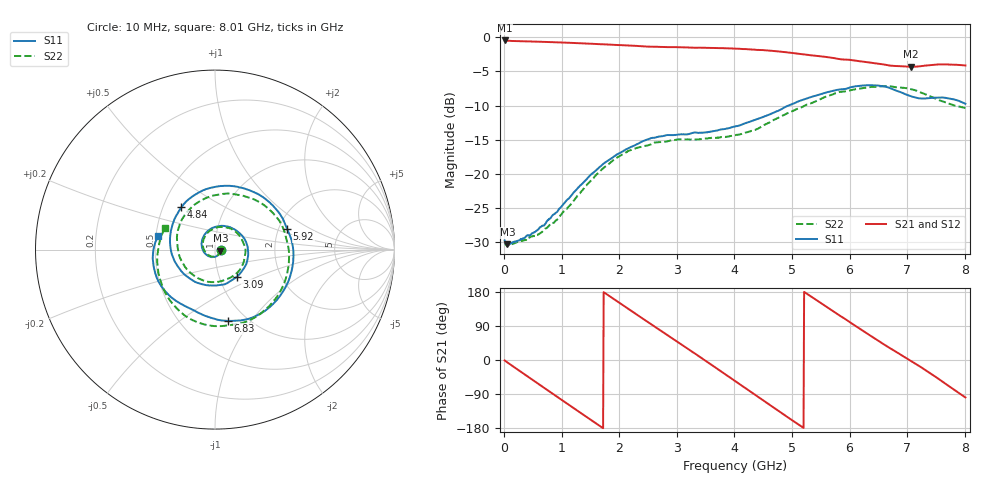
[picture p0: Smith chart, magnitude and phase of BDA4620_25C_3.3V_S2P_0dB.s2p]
!Agilent Technologies,E5071B,MY42404982,A.09.10
!Date: Wed May 06 08:55:57 2026
!Data & Calibration Information:
!Freq	S11:SOLT2(ON)	S21:SOLT2(ON)	S12:SOLT2(ON)	S22:SOLT2(ON)
# Hz S RI R 50
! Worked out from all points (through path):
!   801 points, 10 MHz to 8.01 GHz, reference 50 ohm
!   highest |S21| = -0.45 dB at 10 MHz (marker M1); lowest = -4.3 dB at 7.06 GHz (marker M2)
!   group delay of S21, straight-line fit = 284 ps
!   lowest |S11| = -30.4 dB at 60 MHz (marker M3), VSWR 1.06, Z = 53.1 - j0.535 ohm
!   |S11| at or under -10 dB: start of sweep to 4.939 GHz
!   |S22| runs from -30.6 to -7.2 dB; largest |S21 - S12| = 0.0038
!   S11 on the Smith chart (normalised r, x): 10 MHz: 1.07, -0.01; 3.09 GHz: 1.21, -0.38; 4.84 GHz: 0.62, +0.32; 5.92 GHz: 2.23, +0.62; 6.83 GHz: 0.82, -0.78; 8.01 GHz: 0.51, +0.09
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1e7  0.0323 -0.00235  0.9491 -0.0202  0.9503 -0.0203  0.031 -0.00188
6e7  0.0299 -0.00504  0.9385 -0.1086  0.9405 -0.1101  0.0293 -0.00322
3.6e8  0.0228 -0.025  0.7354 -0.5785  0.7361 -0.5797  0.0245 -0.0213
7.3e8  -0.0134 -0.0417  0.2086 -0.9018  0.2083 -0.9027  -0.00647 -0.0392
1.03e9  -0.0558 -0.0213  -0.2873 -0.8696  -0.2886 -0.8704  -0.047 -0.0231
1.35e9  -0.0743 0.0391  -0.7098 -0.5612  -0.7101 -0.5619  -0.0679 0.0315
1.93e9  0.0308 0.1321  -0.8188 0.324  -0.8196 0.3247  0.0248 0.1258
2.32e9  0.1394 0.0893  -0.4094 0.7617  -0.411 0.7627  0.129 0.0865
2.68e9  0.1854 -0.0246  0.1221 0.8437  0.123 0.8441  0.1694 -0.0122
3.09e9  0.1199 -0.1527  0.6484 0.5428  0.6501 0.5424  0.1228 -0.1296
3.54e9  -0.0286 -0.2  0.832 -0.0929  0.8327 -0.094  -0.013 -0.1811
4.01e9  -0.184 -0.1239  0.471 -0.6797  0.4707 -0.6808  -0.1597 -0.106
4.42e9  -0.2503 0.039  -0.1133 -0.8018  -0.1151 -0.8015  -0.2111 0.0435
4.84e9  -0.1871 0.2364  -0.617 -0.4809  -0.618 -0.481  -0.1378 0.2285
5.35e9  0.0997 0.3538  -0.7136 0.1838  -0.7142 0.1846  0.1281 0.3051
5.92e9  0.4024 0.1145  -0.2167 0.6519  -0.2173 0.6529  0.3952 0.0697
6.27e9  0.4165 -0.1555  0.1912 0.633  0.1917 0.633  0.3921 -0.1695
6.68e9  0.1826 -0.3871  0.5208 0.3404  0.5228 0.3413  0.1932 -0.3935
6.83e9  0.0727 -0.3972  0.5806 0.2048  0.5822 0.2043  0.084 -0.4208
7.06e9  -0.0648 -0.3651  0.6091 -0.0235  0.6111 -0.0242  -0.0882 -0.4079
7.61e9  -0.3102 -0.1858  0.3456 -0.531  0.3457 -0.5321  -0.316 -0.1256
8.01e9  -0.3166 0.0775  -0.0953 -0.6146  -0.0952 -0.6158  -0.2773 0.1215
